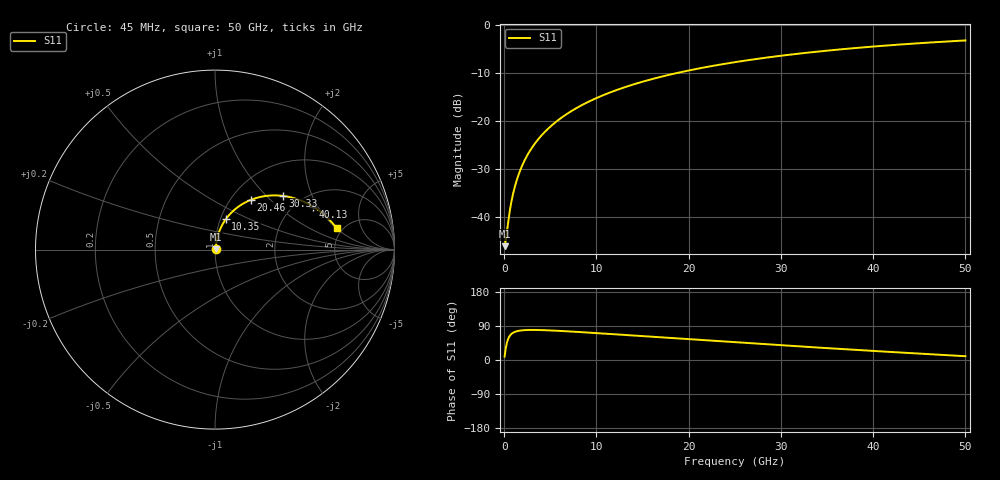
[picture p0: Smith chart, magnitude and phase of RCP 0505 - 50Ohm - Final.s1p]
!Vishay Electro-Films Inc.
!RCP Family
!Case Size 0505
!Assembly Style Surface Mount
!11/2/2015
!efi@vishay.com
# GHz S MA R 50
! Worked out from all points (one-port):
!   801 points, 45 MHz to 50 GHz, reference 50 ohm
!   lowest |S11| = -46.0 dB at 45 MHz (marker M1), VSWR 1.01, Z = 50.5 + j0.0791 ohm
!   |S11| at or under -10 dB: start of sweep to 18.76 GHz
!   S11 on the Smith chart (normalised r, x): 45 MHz: 1.01, +0.00; 10.35 GHz: 1.06, +0.37; 20.46 GHz: 1.23, +0.78; 30.33 GHz: 1.61, +1.25; 40.13 GHz: 2.44, +1.82; 50 GHz: 4.45, +2.02
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0.045  0.005037 8.9
0.1074438  0.00532 20.6
0.2323312  0.006432 38.9
0.6694375  0.01276 65.9
0.794325  0.0148 69.0
0.9816563  0.01793 72.2
1.231431  0.02217 74.9
1.481206  0.02646 76.6
1.730981  0.03077 77.7
2.0432  0.03618 78.5
2.417863  0.0427 79.1
2.854969  0.0503 79.4
3.791625  0.06662 79.1
4.915612  0.08617 78.1
6.289375  0.11 76.5
8.162688  0.1422 73.8
10.34822  0.1794 70.5
12.53375  0.216 67.0
15.46861  0.2641 62.2
18.77812  0.3165 56.9
20.46411  0.3424 54.1
25.0225  0.4094 46.8
30.33022  0.4814 38.5
31.26687  0.4934 37.0
37.51125  0.5677 27.6
40.13389  0.596 23.8
43.75563  0.6323 18.6
50  0.6877 10.0
